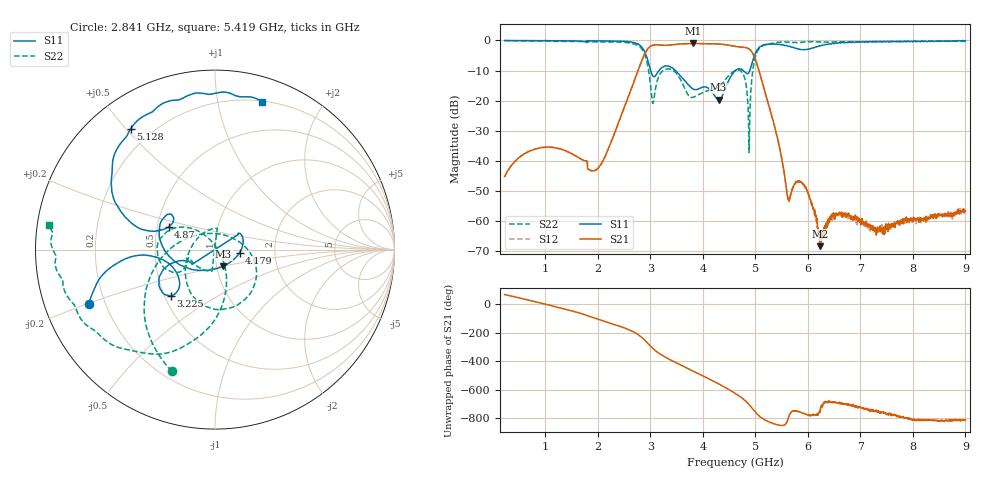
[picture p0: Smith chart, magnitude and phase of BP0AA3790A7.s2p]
!Agilent Technologies,E8358A,US41080443,A.07.50.56
!Agilent E8358A: A.07.50.56
!Date: Wednesday, May 23, 2018 14:52:39
!Correction: S11(Full 2 Port(1,2))
!S21(Full 2 Port(1,2))
!S12(Full 2 Port(1,2))
!S22(Full 2 Port(1,2))
!S2P File: Measurements: S11, S21, S12, S22:
# Hz S  dB  R 50
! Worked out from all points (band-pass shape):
!   1601 points, 225 MHz to 9 GHz, reference 50 ohm
!   highest |S21| = -0.98 dB at 3.817 GHz (marker M1); lowest = -68.4 dB at 6.225 GHz (marker M2)
!   |S21| within 3 dB of the highest: 2.909 GHz to 4.94 GHz (2.031 GHz wide, 51.8 % of centre)
!   lowest |S11| = -19.8 dB at 4.3 GHz (marker M3), VSWR 1.23, Z = 53.8 - j10 ohm
!   |S11| at or under -10 dB: 3.007 GHz to 3.164 GHz (157.7 MHz wide, 5.11 % of centre); 3.478 GHz to 4.617 GHz (1.139 GHz wide, 28.1 % of centre); 4.77 GHz to 4.894 GHz (124 MHz wide, 2.57 % of centre)
!   |S22| runs from -37.3 to 0.0 dB; largest |S21 - S12| = 0.0079
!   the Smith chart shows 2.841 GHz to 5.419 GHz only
!   S11 on the Smith chart (normalised r, x): 2.841 GHz: 0.14, -0.20; 3.225 GHz: 0.54, -0.32; 4.179 GHz: 1.32, -0.05; 4.87 GHz: 0.57, +0.16; 5.128 GHz: 0.13, +0.51; 5.419 GHz: 0.21, +1.35
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2.25e8  -0.02 -7.7  -45.26 69.1  -45.30 68.8  -0.08 -31.3
8.063438e8  -0.05 -29.0  -36.11 18.8  -36.17 18.7  -0.22 -113.0
1.245094e9  -0.11 -48.3  -35.89 -21.4  -35.94 -21.7  -0.30 -175.4
1.689328e9  -0.34 -78.3  -39.58 -65.2  -39.58 -65.5  -0.30 125.4
2.287125e9  -0.19 -92.9  -32.26 -138.7  -32.33 -138.9  -0.57 6.5
2.841047e9  -2.33 -156.8  -6.59 126.4  -6.58 126.5  -2.87 -109.5
3.043969e9  -11.74 -159.2  -1.59 51.3  -1.62 51.4  -20.84 95.9
3.153656e9  -10.24 -132.3  -1.45 18.2  -1.53 18.3  -12.29 -21.3
3.224953e9  -8.96 -134.0  -1.56 1.0  -1.61 1.2  -10.30 -47.2
3.817266e9  -16.19 -153.2  -0.98 -111.3  -1.03 -111.2  -18.89 111.3
4.179234e9  -17.21 -7.1  -1.11 -176.0  -1.13 -176.1  -16.27 -162.9
4.299891e9  -19.75 -63.8  -1.19 160.8  -1.19 160.9  -15.53 -156.1
4.6125e9  -10.08 169.3  -1.96 94.3  -2.02 94.4  -10.12 -166.6
4.870266e9  -10.82 153.7  -2.71 18.5  -2.75 18.6  -27.02 110.1
5.128031e9  -1.73 125.0  -13.69 -82.0  -13.76 -82.3  -1.90 -144.6
5.418703e9  -1.27 72.3  -32.34 -128.1  -32.25 -127.7  -0.60 171.6
5.621625e9  -1.94 31.7  -52.82 -89.3  -52.91 -85.3  -0.51 153.6
5.758734e9  -2.58 -5.9  -47.46 -31.4  -47.48 -31.0  -0.63 143.7
6.076828e9  -2.57 -117.8  -54.20 -56.7  -54.52 -60.0  -0.34 120.2
6.224906e9  -1.82 -155.8  -68.45 -28.2  -65.74 -29.8  -0.49 111.0
7.541156e9  -0.48 99.0  -61.76 -58.8  -62.60 -54.3  -0.42 29.9
9e9  -0.11 60.5  -56.83 -94.5  -56.42 -93.7  -0.30 -16.8
